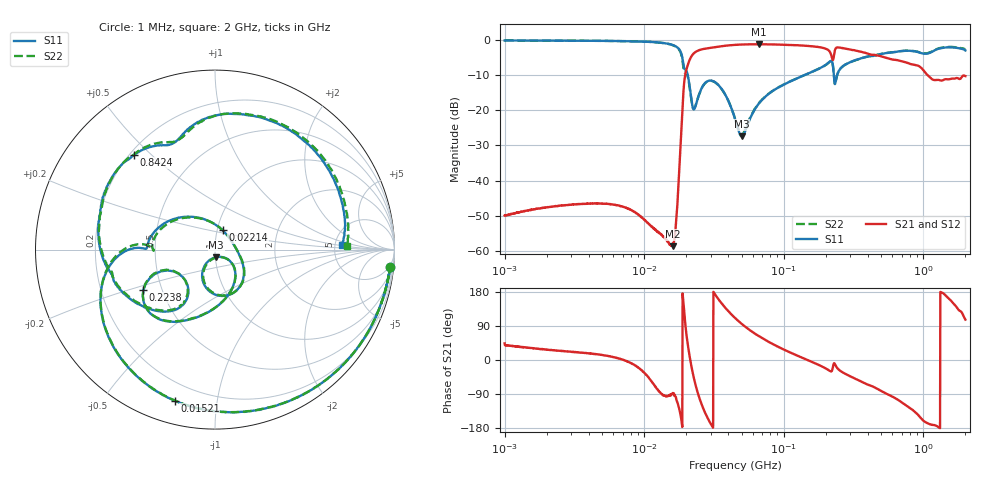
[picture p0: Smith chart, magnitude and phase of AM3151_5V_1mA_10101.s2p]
! Date/Time: Fri Jun 26 11:00:00 2020
! Network Analyzer:  Rev:
! Sweep from 1000000.0 to 2000000000.0, 1601 Points ! Power Supply: 0 V, 0 A
# HZ S DB R 50
!freq MagS11 AngS11 MagS21 AngS21 MagS12 AngS12 MagS22 AngS22
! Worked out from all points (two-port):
!   1601 points, 1 MHz to 2 GHz, reference 50 ohm
!   highest |S21| = -1.24 dB at 66.65 MHz (marker M1); lowest = -58.6 dB at 16.03 MHz (marker M2)
!   |S21| within 3 dB of the highest: 22.18 MHz to 218.3 MHz (196.2 MHz wide, 163 % of centre); 229.1 MHz to 428 MHz (198.9 MHz wide, 60.5 % of centre)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
!   lowest |S11| = -27.4 dB at 49.88 MHz (marker M3), VSWR 1.09, Z = 50.5 - j4.24 ohm
!   |S11| at or under -10 dB: 20.5 MHz to 140.8 MHz (120.3 MHz wide, 149 % of centre); 228.4 MHz to 241.2 MHz (12.78 MHz wide, 5.44 % of centre)
!   |S22| runs from -26.9 to -0.2 dB; largest |S21 - S12| = 0.0078
!   S11 on the Smith chart (normalised r, x): 1 MHz: 4, -19; 15.21 MHz: 0.11, -0.76; 22.14 MHz: 1.06, +0.23; 223.8 MHz: 0.39, -0.22; 842.4 MHz: 0.22, +0.44; 2 GHz: 5.77, +0.64
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1000000  -0.17 -5.8  -49.93 43.9  -49.96 38.8  -0.17 -5.8
3555161  -0.25 -19.7  -46.61 19.6  -46.62 19.2  -0.24 -19.6
7748448  -0.37 -44.0  -48.06 -5.3  -48.04 -5.6  -0.38 -44.1
1.263916e7  -0.73 -79.0  -54.73 -80.3  -54.60 -80.9  -0.74 -79.4
1.521181e7  -1.20 -105.0  -58.09 -93.7  -58.22 -93.0  -1.22 -105.8
1.602785e7  -1.47 -115.7  -58.64 -86.9  -58.80 -86.6  -1.51 -116.8
1.70489e7  -1.97 -132.2  -50.31 -106.0  -50.46 -104.5  -2.05 -133.9
1.947442e7  -8.30 179.4  -11.08 114.8  -11.09 114.8  -9.36 -179.4
2.051914e7  -10.07 151.3  -7.13 41.1  -7.13 41.0  -10.38 152.1
2.213957e7  -18.75 68.7  -4.28 -29.5  -4.28 -29.5  -18.81 65.8
2.481331e7  -15.35 -26.1  -2.90 -99.6  -2.89 -99.6  -15.36 -25.0
2.986397e7  -11.56 -75.0  -2.25 -167.4  -2.25 -167.3  -11.59 -73.2
4.493426e7  -22.74 -119.9  -1.41 110.3  -1.41 110.2  -22.63 -116.5
4.988463e7  -27.45 -80.9  -1.32 95.5  -1.32 95.5  -26.90 -78.7
6.66528e7  -17.96 -39.6  -1.24 62.3  -1.26 62.3  -17.87 -39.7
1.589914e8  -9.09 -96.3  -1.82 -5.0  -1.81 -5.1  -9.10 -96.5
2.238309e8  -6.78 -150.6  -5.71 -22.2  -5.71 -22.3  -6.77 -150.5
2.449739e8  -9.25 -119.8  -2.15 -23.9  -2.15 -23.8  -9.27 -120.7
5.652395e8  -3.63 171.3  -5.31 -92.0  -5.28 -92.0  -3.64 169.2
8.424353e8  -3.17 130.5  -6.99 -132.5  -6.95 -132.5  -3.15 128.1
1.413901e9  -2.20 72.8  -11.26 173.5  -11.24 173.6  -2.11 70.0
2e9  -3.00 2.2  -10.31 106.7  -10.46 106.2  -2.66 1.5
